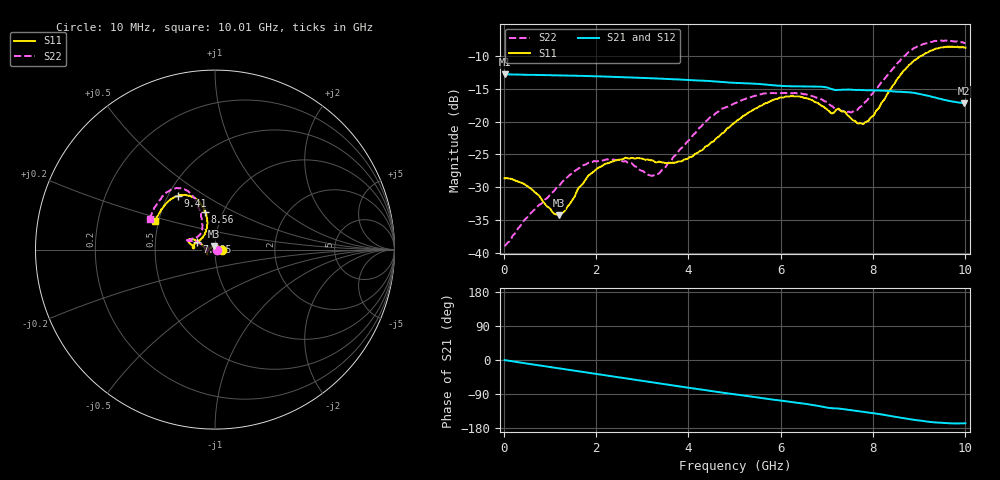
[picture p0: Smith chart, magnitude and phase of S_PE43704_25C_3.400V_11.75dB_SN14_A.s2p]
! Device ID: PE43704
! Dir: z:\PE43704\PE43704_Char_1_20130516\PE43704\AMB\3p400V\11p75dB
! Serial: 14
! Insertion: A
! Impedance: 50 ohm
! Temp: Amb
! VDD: 3.400V
! Attenuation Step: 11.75dB
! IDD: 1.139902e-01mA
#  Hz  S  RI  R  50
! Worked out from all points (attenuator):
!   401 points, 10 MHz to 10.01 GHz, reference 50 ohm
!   highest |S21| = -12.76 dB at 10 MHz (marker M1); lowest = -17.2 dB at 9.985 GHz (marker M2)
!   lowest |S11| = -34.3 dB at 1.185 GHz (marker M3), VSWR 1.04, Z = 49.1 + j1.71 ohm
!   |S11| at or under -10 dB: start of sweep to 9.031 GHz
!   |S22| runs from -39.0 to -7.6 dB; largest |S21 - S12| = 0.0017
!   S11 on the Smith chart (normalised r, x): 10 MHz: 1.08, +0.00; 7.485 GHz: 0.81, +0.07; 8.56 GHz: 0.82, +0.37; 9.41 GHz: 0.56, +0.39; 10.01 GHz: 0.48, +0.18
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1e7  0.037 0.000287  0.2302 -0.000838  0.2302 -0.000813  0.0112 0.000339
4.85e8  0.0276 0.0172  0.2255 -0.0366  0.2254 -0.0365  0.00376 0.018
1.185e9  -0.00835 0.0174  0.2094 -0.0856  0.2094 -0.0854  -0.0278 0.0165
1.685e9  -0.0328 9.12e-06  0.1912 -0.1167  0.1912 -0.1166  -0.046 -0.00186
2.01e9  -0.0419 -0.0121  0.1767 -0.1348  0.1768 -0.1347  -0.048 -0.0133
2.41e9  -0.0449 -0.0232  0.1567 -0.1546  0.1567 -0.1545  -0.047 -0.0202
3.135e9  -0.0434 -0.0272  0.1148 -0.182  0.1149 -0.182  -0.0379 -0.0101
3.36e9  -0.0441 -0.0226  0.101 -0.1882  0.1013 -0.1881  -0.0402 -0.00283
4.035e9  -0.0537 0.00119  0.0581 -0.1995  0.0584 -0.1996  -0.0701 0.0229
4.46e9  -0.065 0.0186  0.031 -0.2023  0.0312 -0.2024  -0.0977 0.0449
5.01e9  -0.0899 0.0408  -0.00199 -0.1983  -0.00188 -0.1983  -0.1301 0.0475
5.96e9  -0.1393 0.0588  -0.0532 -0.1807  -0.0526 -0.1808  -0.1585 0.0469
6.685e9  -0.1417 0.0356  -0.0886 -0.1633  -0.0889 -0.1632  -0.149 0.0495
7.085e9  -0.1159 0.0163  -0.1074 -0.143  -0.1076 -0.1435  -0.1173 0.0627
7.485e9  -0.1017 0.0412  -0.1173 -0.1311  -0.1169 -0.1315  -0.0869 0.0816
7.86e9  -0.0635 0.0771  -0.1292 -0.1168  -0.1289 -0.1173  -0.0713 0.1245
8.36e9  -0.0437 0.1656  -0.1443 -0.093  -0.1439 -0.0933  -0.0849 0.2198
8.56e9  -0.0546 0.2116  -0.1494 -0.0806  -0.1486 -0.0809  -0.1046 0.2663
8.935e9  -0.103 0.2806  -0.1538 -0.0604  -0.1534 -0.0587  -0.1631 0.3319
9.41e9  -0.2066 0.2978  -0.146 -0.0385  -0.1459 -0.0382  -0.2547 0.3257
9.985e9  -0.327 0.1685  -0.135 -0.0306  -0.1359 -0.0303  -0.3578 0.178
1.001e10  -0.3322 0.1589  -0.1354 -0.0313  -0.136 -0.0313  -0.3619 0.1697
